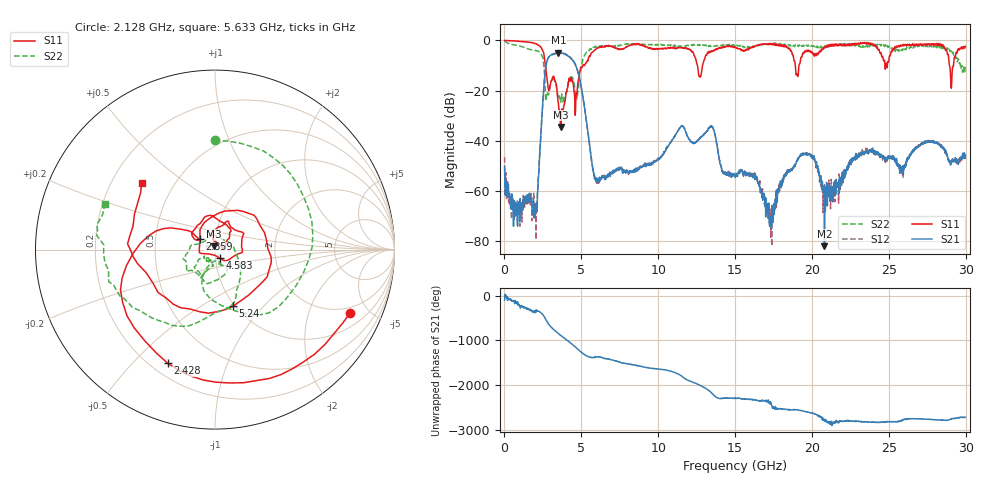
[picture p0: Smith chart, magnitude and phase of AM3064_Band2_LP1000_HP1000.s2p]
# Hz S DB R 50.0
!freq dBS11 angS11 dBS21 angS21 dBS12 angS12 dBS22 angS22
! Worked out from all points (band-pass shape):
!   1600 points, 10 MHz to 29.98 GHz, reference 50 ohm
!   highest |S21| = -4.88 dB at 3.515 GHz (marker M1); lowest = -82.0 dB at 20.82 GHz (marker M2)
!   |S21| within 3 dB of the highest: 2.79 GHz to 4.435 GHz (1.646 GHz wide, 45.6 % of centre)
!   lowest |S11| = -34.5 dB at 3.665 GHz (marker M3), VSWR 1.04, Z = 49.5 + j1.8 ohm
!   |S11| at or under -10 dB: 2.667 GHz to 5.093 GHz (2.426 GHz wide, 62.5 % of centre); 12.55 GHz to 12.89 GHz (335.6 MHz wide, 2.64 % of centre); 28.95 GHz to 29.2 GHz (258 MHz wide, 0.887 % of centre)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
!   |S22| runs from -24.7 to -0.3 dB; largest |S21 - S12| = 0.013
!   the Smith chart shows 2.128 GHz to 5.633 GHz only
!   S11 on the Smith chart (normalised r, x): 2.128 GHz: 1.67, -3.81; 2.428 GHz: 0.27, -0.63; 2.859 GHz: 0.84, +0.10; 4.583 GHz: 1.05, -0.10; 5.24 GHz: 0.98, -0.69; 5.633 GHz: 0.33, +0.35
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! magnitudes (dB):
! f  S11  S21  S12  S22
! 10 MHz  0.0  -50.3  -46.5  -0.3
! 703.5 MHz  -0.2  -66.6  -65.1  -1.9
! 2.128 GHz  -1.6  -67.1  -63.4  -4.3
! 2.428 GHz  -3.3  -31.3  -31.2  -6.1
! 2.859 GHz  -19.7  -6.9  -6.9  -21.7
! 3.515 GHz  -25.6  -4.9  -4.9  -23.2
! 3.665 GHz  -34.5  -5.1  -5.0  -24.2
! 4.583 GHz  -25.1  -9.5  -9.4  -20.4
! 5.015 GHz  -10.9  -19.5  -19.4  -9.5
! 5.24 GHz  -9.6  -28.2  -28.1  -5.7
! 5.633 GHz  -5.2  -46.4  -46.5  -3.6
! 6.083 GHz  -3.1  -55.6  -56.1  -2.6
! 10 GHz  -3.4  -47.6  -47.2  -1.8
! 13.43 GHz  -4.7  -34.1  -34.1  -2.3
! 15 GHz  -2.6  -53.5  -54.1  -1.9
! 16.3 GHz  -2.2  -53.8  -54.0  -2.3
! 17.33 GHz  -1.4  -71.9  -78.4  -1.4
! 19.99 GHz  -4.7  -46.2  -46.2  -2.0
! 20.82 GHz  -2.8  -82.0  -57.4  -2.4
! 25 GHz  -8.3  -47.0  -45.6  -2.2
! 29.08 GHz  -17.7  -48.2  -48.8  -5.1
! 29.98 GHz  -2.4  -45.9  -45.2  -10.5
